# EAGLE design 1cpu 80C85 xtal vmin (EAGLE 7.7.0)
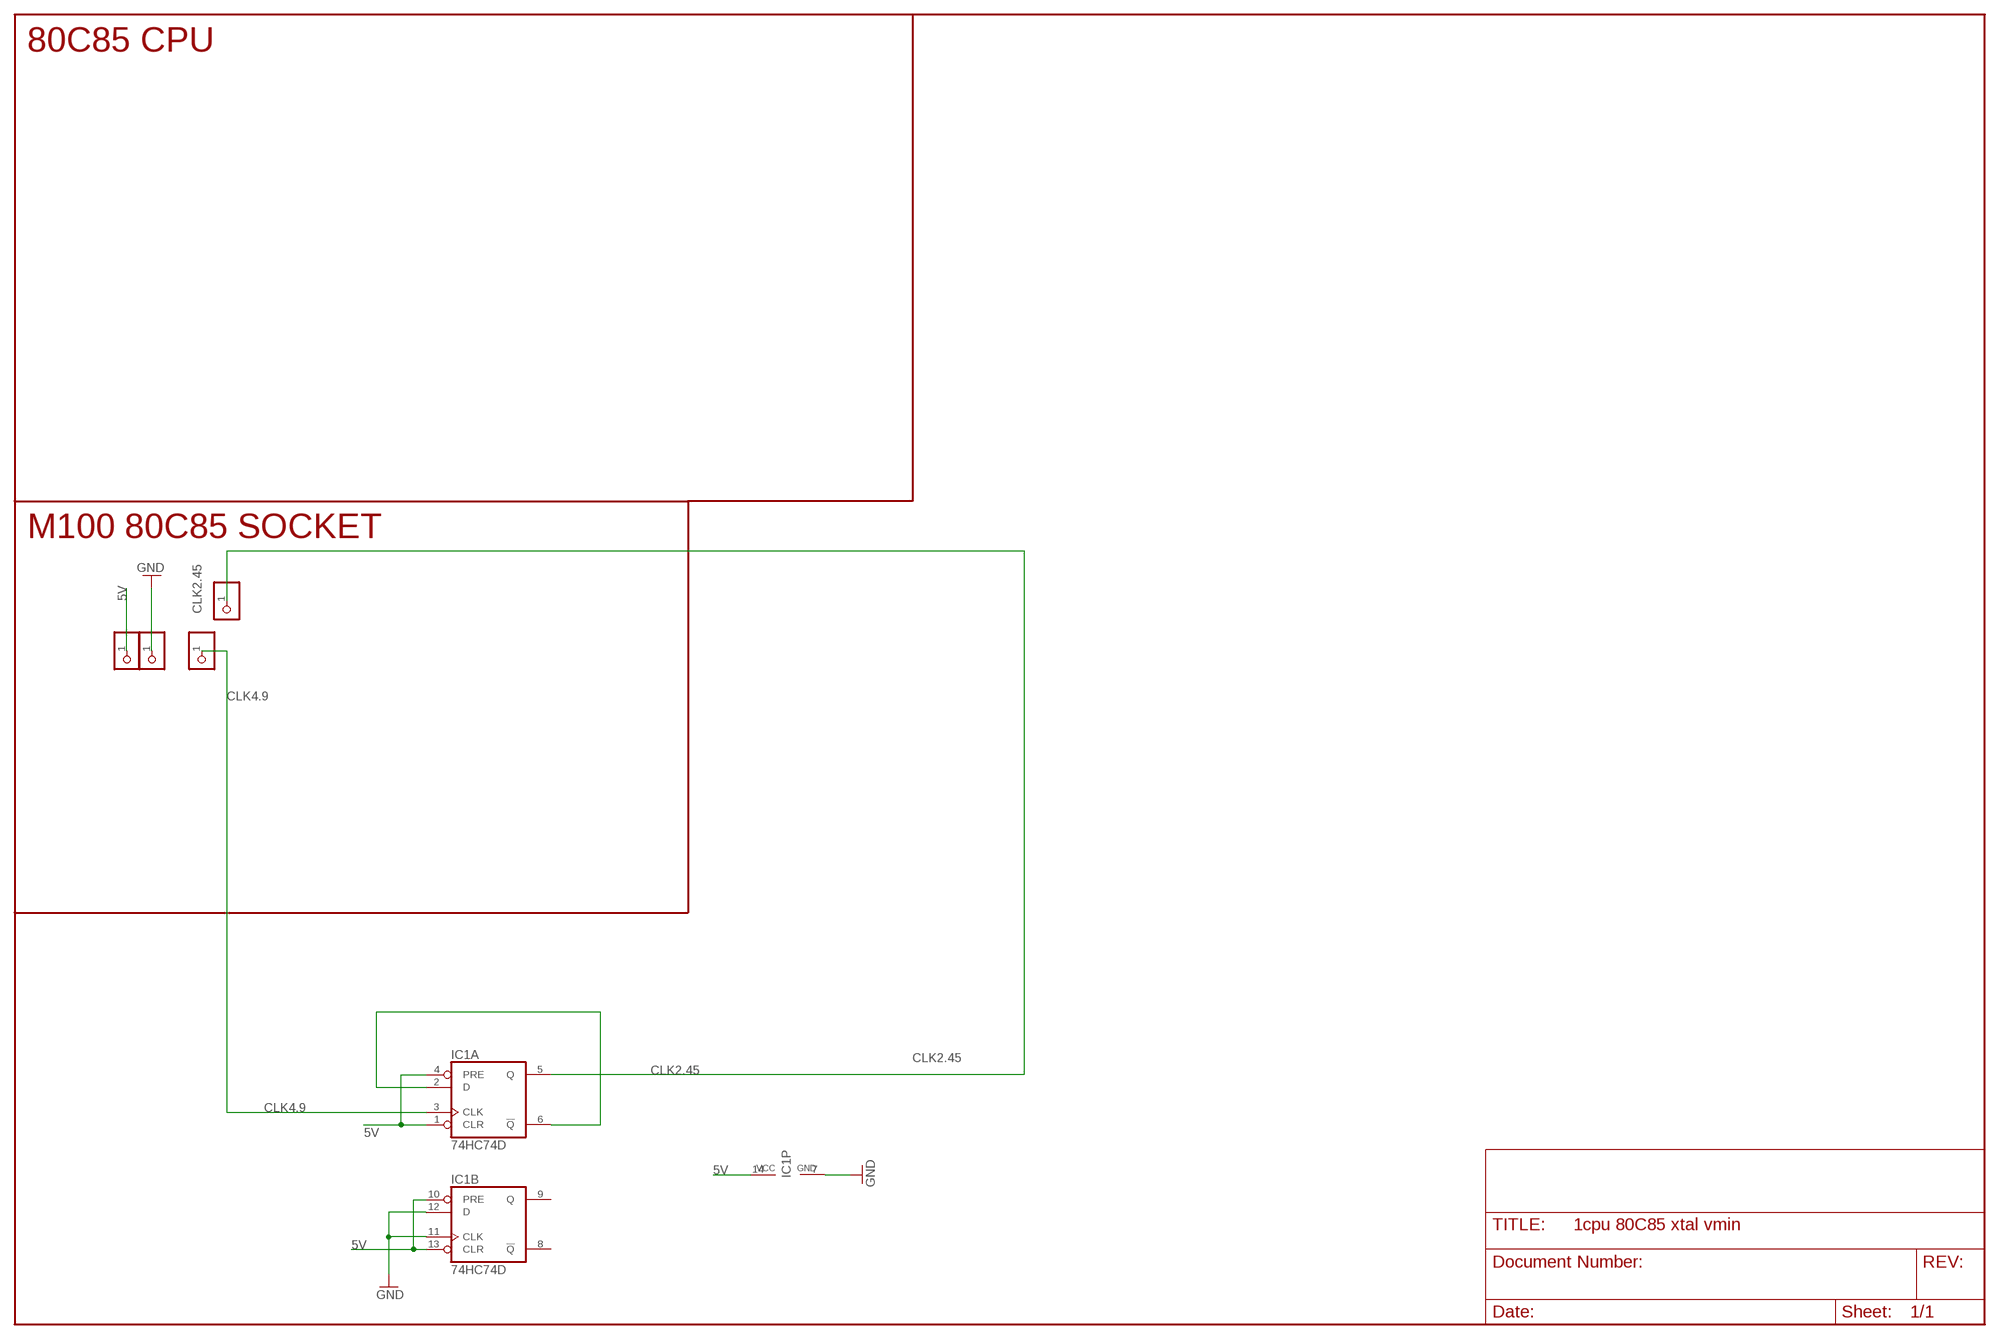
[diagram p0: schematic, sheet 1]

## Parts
5V  PINHD-1X1  [1X01]
GND  PINHD-1X1  [1X01]
IC1  74HC74D  [SO14]
SEL1  PINHD-1X1  [1X01]
SEL2  PINHD-1X1  [1X01]

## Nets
5V: 5V.1 IC1.1(A:CLR) IC1.4(A:PRE) IC1.10(B:PRE) IC1.13(B:CLR) IC1.14(P:VCC)
CLK2.45: IC1.5(A:Q) SEL2.1
CLK4.9: IC1.3(A:CLK) SEL1.1
GND: GND.1 IC1.7(P:GND) IC1.11(B:CLK) IC1.12(B:D)
N$2: IC1.2(A:D) IC1.6(A:!Q)
Unconnected: IC1.8(B:!Q) IC1.9(B:Q)

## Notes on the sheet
- 80C85 CPU
- M100 80C85 SOCKET

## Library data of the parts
5V GND SEL1 SEL2 = pinhead:PINHD-1X1: PIN HEADER
IC1 = 74xx-eu:74*74: Dual D type positive edge triggered FLIP FLOP, preset and clear

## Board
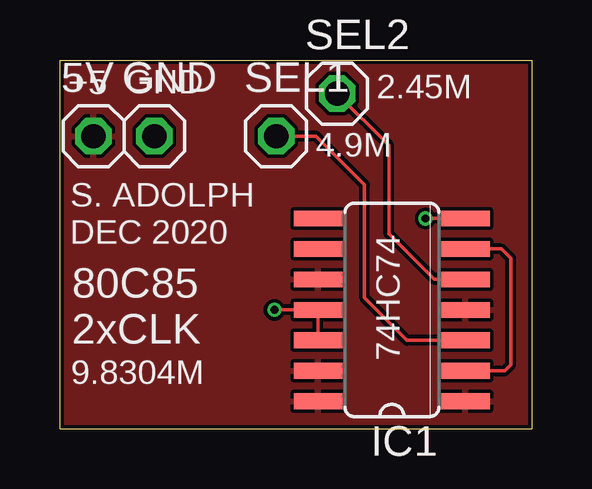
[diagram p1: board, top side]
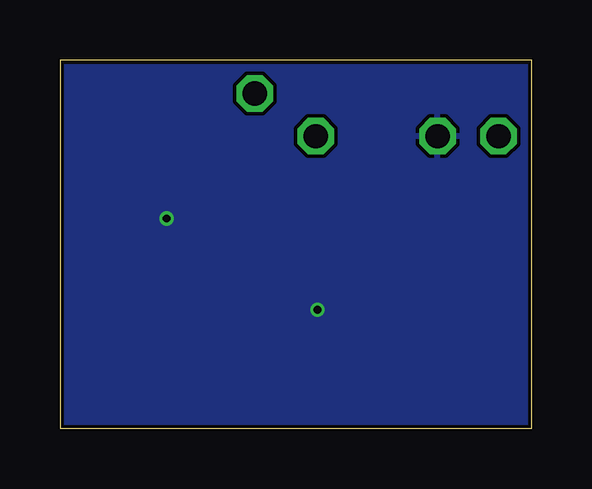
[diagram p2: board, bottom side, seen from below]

Size 19.68 x 15.37 mm. Coordinates in mm from the lower left corner, seen from the top.
Outline: 0,0 19.68,0 19.68,15.37 0,15.37 0,0
Copper layers (1*16): Top 0.035559375mm / dielectric 1.6mm / Bottom 0.035559375mm
Design rules "oshpark-2layer *": minimum track width 6mil, minimum drill 10mil, track to track 6mil, track to pad 6mil, pad to pad 6mil, via to via 6mil, smd to smd 6mil, copper to edge 6mil, drill to drill 6mil, minimum pad ring 5mil, minimum via ring 5mil, stop-mask expansion 2.5mil, vias tented up to drill 0mil, thermal gap 6mil

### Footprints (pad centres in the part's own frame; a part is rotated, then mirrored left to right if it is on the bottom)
1X01 = drill 1.016 octagon: 1 0,0
SO14 = smd 0.66 x 2.032: 1 -3.81,-3.073; 2 -2.54,-3.073; 3 -1.27,-3.073; 4 0,-3.073; 5 1.27,-3.073; 6 2.54,-3.073; 7 3.81,-3.073; 8 3.81,3.073; 9 2.54,3.073; 10 1.27,3.073; 11 0,3.073; 12 -1.27,3.073; 13 -2.54,3.073; 14 -3.81,3.073

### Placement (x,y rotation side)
5V  1.4,12.19 0 top
GND  3.94,12.19 0 top
IC1  13.84,4.95 90 top
SEL1  9.02,12.19 0 top
SEL2  11.56,13.97 0 top

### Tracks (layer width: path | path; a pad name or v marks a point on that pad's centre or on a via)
5V
  pour Top: 0.08,15.29 0.08,0.09 19.61,0.08 19.61,15.29
CLK2.45
  Top 0.152: IC1.5 15.62,6.22 13.72,8.13 13.72,11.81 SEL2.1
CLK4.9
  Top 0.152: IC1.3 14.48,3.68 12.7,5.46 12.7,10.16 10.67,12.19 SEL1.1
GND  (via drill 0.33)
  Top 0.152: IC1.7 v15.24,8.76 | v8.94,4.95 IC1.11 IC1.12
  Bottom 0.152: v15.24,8.76 15.29,8.76 | v8.94,4.95 8.84,4.95 8.83,4.97
  pour Bottom: 0.08,15.29 19.61,15.29 19.61,0.08 0.08,0.09
N$2
  Top 0.152: IC1.2 18.54,2.41 18.8,2.67 18.8,7.11 18.41,7.49 IC1.6

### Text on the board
_tsilk: +5 | GND | 2.45M | 4.9M | S. ADOLPH | DEC 2020 | 74HC74 | 80C85 / 2xCLK | 9.8304M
